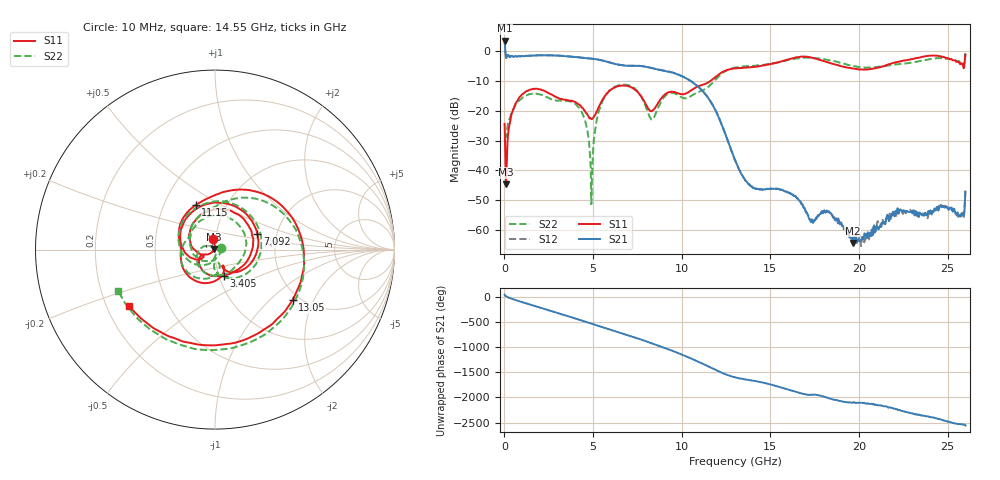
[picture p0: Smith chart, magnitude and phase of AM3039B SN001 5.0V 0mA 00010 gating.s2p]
!Agilent Technologies,E8364B,MY43040894,A.07.50.67
!Agilent E8364B: A.07.50.67
!Date: Tuesday, June 28, 2016 08:03:49
!Correction: S11(Full 2 Port(1,2))
!S21(Full 2 Port(1,2))
!S12(Full 2 Port(1,2))
!S22(Full 2 Port(1,2))
!S2P File: Measurements: S11, S21, S12, S22:
# Hz S  dB  R 50
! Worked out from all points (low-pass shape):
!   1601 points, 10 MHz to 26 GHz, reference 50 ohm
!   highest |S21| = 3.55 dB at 10 MHz (marker M1); lowest = -64.4 dB at 19.65 GHz (marker M2)
!   |S21| within 3 dB of the highest: start of sweep to 44.76 MHz
!   lowest |S11| = -44.8 dB at 91.22 MHz (marker M3), VSWR 1.01, Z = 49.5 + j0.178 ohm
!   |S11| at or under -10 dB: start of sweep to 11.62 GHz
!   |S22| runs from -51.4 to -0.8 dB; largest |S21 - S12| = 0.024
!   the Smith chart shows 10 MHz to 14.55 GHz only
!   S11 on the Smith chart (normalised r, x): 10 MHz: 0.97, +0.11; 3.405 GHz: 1.06, -0.31; 7.092 GHz: 1.58, +0.30; 11.15 GHz: 0.72, +0.39; 13.05 GHz: 1.84, -1.40; 14.55 GHz: 0.29, -0.27
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1e7  -24.41 102.4  3.55 40.5  3.60 41.3  -29.85 11.4
9.121875e7  -44.77 161.9  -2.21 4.8  -2.11 4.7  -28.53 -59.3
7.572125e8  -16.40 158.2  -1.74 -83.6  -1.69 -83.4  -17.18 171.9
1.650619e9  -12.64 66.2  -1.47 -179.9  -1.43 -179.8  -14.15 69.8
2.511538e9  -14.13 -11.6  -1.40 87.9  -1.34 87.9  -15.77 -10.4
3.404944e9  -16.27 -70.6  -1.66 -9.4  -1.61 -9.3  -16.69 -76.1
4.347081e9  -18.80 -140.4  -2.18 -113.0  -2.16 -112.9  -20.34 -171.2
4.915612e9  -22.80 -152.2  -2.53 -176.6  -2.50 -176.6  -50.23 -108.2
5.662825e9  -15.09 -179.9  -3.33 97.6  -3.29 97.7  -15.34 -165.5
7.092275e9  -11.96 20.5  -4.92 -59.5  -4.88 -59.4  -11.63 8.7
8.684162e9  -17.27 -69.7  -6.20 106.8  -6.14 106.9  -18.79 -79.0
1.115321e10  -11.35 113.3  -13.21 111.4  -13.19 111.2  -13.20 102.9
1.3005e10  -5.81 -28.8  -36.57 -162.7  -36.54 -163.1  -5.48 -35.8
1.305373e10  -5.76 -32.9  -37.29 -167.1  -37.24 -166.9  -5.42 -40.1
1.454816e10  -4.84 -147.0  -46.67 93.8  -46.44 93.5  -4.64 -156.8
1.617253e10  -2.50 83.4  -48.09 -62.4  -47.90 -64.0  -2.76 79.8
1.734208e10  -2.18 -27.7  -56.48 -147.5  -57.25 -148.1  -2.22 -19.2
1.964869e10  -5.80 146.6  -64.43 60.3  -63.54 60.5  -4.92 156.4
2.167916e10  -4.38 11.8  -56.94 -43.1  -55.97 -37.1  -4.79 17.0
2.416446e10  -1.47 178.9  -53.66 120.2  -54.16 121.6  -2.50 -166.9
2.513908e10  -2.64 95.4  -52.65 30.0  -52.88 22.4  -2.67 111.4
2.6e10  -1.17 -25.8  -47.29 -38.3  -46.78 -39.6  -0.75 1.3
